| IBIS file nevis_100lqfp_derated.ibs generated by Daphne version: 2018.03.27
[IBIS Ver]   5.0
[Comment Char]   |_char
[File Name]   nevis_100lqfp_derated.ibs
[File Rev]   1
[Date]   Tue Nov  6 17:26:38 2018
[Source]   NXP Viper 2018.03.27
[Notes]
[Disclaimer] IMPORTANT NOTICE
  This information is provided on an AS IS basis and without warranty.
  IN NO EVENT SHALL NXP BE LIABLE FOR INCIDENTAL OR CONSEQUENTIAL
  DAMAGES ARISING FROM USE OF THIS INFORMATION. THIS DISCLAIMER OF
  WARRANTY EXTENDS TO THE USER OF THE INFORMATION, AND TO THEIR CUSTOMERS
  OR USERS OF PRODUCTS  AND IS IN LIEU OF ALL WARRANTIES WHETHER EXPRESS,
  IMPLIED, OR STATUTORY, INCLUDING IMPLIED WARRANTIES OF MERCHANTABILITY
  OR FITNESS FOR PARTICULAR PURPOSE.
  NXP does not represent or warrant that the information furnished
  hereunder is free of infringement of any third party patents,
  copyrights, trade secrets, or other intellectual property rights.
  NXP does not represent or warrant that the information is free of
  defect, or that it meets any particular standard, requirements or need
  of the user of the infomation or their customers.
  NXP reserves the right to change the information in this file
  without notice.
   http://www.nxp.com
[Copyright]   (C) Copyright NXP 2004 - 2018, All Rights Reserved.
|   NEVIS:100LQFP
[Component]   NEVIS:100LQFP
[Manufacturer]   NXP
[Package]
| variable   typ   min   max
R_pkg   0.12938   0.084596   0.14923
L_pkg   4.494e-09   3.339e-09   5.624e-09
C_pkg   9.253e-13   7.884e-13   1.210e-12
[Pin] signal_name   model_name   R_pin   L_pin   C_pin
1   TCK   p_io_5vtol_4m   0.13839   5.358e-09 9.081e-13
2   RESETB   p_vpp_5vtol_4m   0.084596  4.716e-09 1.210e-12
3   GPIOC0   p_io_5vtol_4m   0.12944   4.882e-09 9.510e-13
4   GPIOC1   p_io_5vtol_4m   0.12633   4.637e-09 9.568e-13
5   GPIOC2   p_io_5vtol_4m   0.12482   4.358e-09 9.723e-13
6   GPIOF8   p_io_5vtol_4m   0.12996   3.587e-09 8.978e-13
7   VDD33   POWER   NA   NA   NA
8   VSS   GND   NA   NA   NA
9   GPIOD6   p_io_5vtol_4m   0.12568   3.453e-09 8.861e-13
10   GPIOD5   p_io_5vtol_4m   0.12166   3.927e-09 8.389e-13
11   GPIOC3   p_io_5vtol_4m   0.11505   3.887e-09 8.150e-13
12   GPIOC4   p_io_5vtol_4m   0.11662   3.982e-09 9.402e-13
13   GPIOA10   p_io_5vtol_4m   0.11619   3.798e-09 7.884e-13
14   GPIOA9   p_io_5vtol_4m   0.12215   3.545e-09 8.020e-13
15   VSS   GND   NA   NA   NA
16   VDD   POWER   NA   NA   NA
17   GPIOA7   p_io_5vtol_4m   0.12328   3.627e-09 8.876e-13
18   GPIOA8   p_io_5vtol_4m   0.12024   4.091e-09 8.720e-13
19   GPIOA6   p_io_5vtol_4m   0.12076   4.379e-09 8.539e-13
20   GPIOA5   p_io_5vtol_4m   0.12153   4.556e-09 9.300e-13
21   GPIOA4   p_io_5vtol_4m   0.12459   4.784e-09 9.582e-13
22   GPIOA0   p_io_5vtol_4m   0.1277   4.982e-09 1.043e-12
23   GPIOA1   p_io_5vtol_4m   0.13134   5.169e-09 9.858e-13
24   GPIOA2   p_io_5vtol_4m   0.13511   5.278e-09 1.058e-12
25   GPIOA3   p_io_5vtol_4m   0.1403   5.579e-09 9.224e-13
26   GPIOB7   p_io_5vtol_4m   0.14428   5.567e-09 8.922e-13
27   GPIOC5   p_io_5vtol_4m   0.086695  4.756e-09 1.146e-12
28   GPIOB6   p_io_5vtol_4m   0.13488   4.874e-09 9.254e-13
29   GPIOB5   p_io_5vtol_4m   0.13539   4.494e-09 9.544e-13
30   GPIOB4   p_io_5vtol_4m   0.14179   3.764e-09 1.043e-12
31   VDDA   POWER   NA   NA   NA
32   VSSA   GND   NA   NA   NA
33   GPIOB0   p_io_5vtol_4m   0.13966   3.558e-09 8.476e-13
34   GPIOB1   p_io_5vtol_4m   0.14138   3.454e-09 8.946e-13
35   VDD   POWER   NA   NA   NA
36   GPIOB2   p_io_5vtol_4m   0.13932   3.570e-09 8.125e-13
37   GPIOA11   p_io_5vtol_4m   0.14249   3.673e-09 9.251e-13
38   VSS_USB   GND   NA   NA   NA
39   USB_DP   NC   0.14676   3.468e-09 8.492e-13
40   USB_DM   NC   0.14622   3.418e-09 9.220e-13
41   VDD_USB   POWER   NA   NA   NA
42   GPIOB3   p_io_5vtol_4m   0.14251   3.392e-09 8.778e-13
43   VDD33   POWER   NA   NA   NA
44   VSS   GND   NA   NA   NA
45   GPIOF11   p_io_5vtol_4m   0.14188   3.731e-09 9.937e-13
46   GPIOF15   p_io_5vtol_4m   0.13496   4.493e-09 9.338e-13
47   GPIOD7   p_io_5vtol_4m   0.13493   4.834e-09 1.059e-12
48   GPIOG11   p_io_5vtol_4m   0.13554   5.103e-09 9.630e-13
49   GPIOC6   p_io_5vtol_4m   0.13844   5.328e-09 1.077e-12
50   GPIOC7   p_io_5vtol_4m   0.14231   5.624e-09 9.638e-13
51   GPIOG10   p_io_5vtol_4m   0.1376   5.575e-09 9.335e-13
52   GPIOC8   p_io_5vtol_4m   0.12912   5.293e-09 1.144e-12
53   GPIOC9   p_io_5vtol_4m   0.12493   5.103e-09 9.020e-13
54   GPIOC10   p_io_5vtol_4m   0.12177   4.924e-09 9.088e-13
55   GPIOF0   p_io_5vtol_4m   0.11876   4.771e-09 9.386e-13
56   GPIOF10   p_io_5vtol_4m   0.1159   4.642e-09 9.030e-13
57   GPIOF9   p_io_5vtol_4m   0.11553   4.566e-09 9.000e-13
58   GPIOC11   p_io_5vtol_4m   0.11627   4.472e-09 8.361e-13
59   GPIOC12   p_io_5vtol_4m   0.11483   4.368e-09 8.595e-13
60   GPIOF2   p_io_5vtol_4m   0.1176   4.372e-09 8.162e-13
61   GPIOF3   p_io_5vtol_4m   0.11313   4.189e-09 8.385e-13
62   GPIOF4   p_io_5vtol_4m   0.11588   4.167e-09 8.970e-13
63   GPIOF5   p_io_5vtol_4m   0.11563   4.018e-09 8.227e-13
64   GPIOG8   p_io_5vtol_4m   0.11982   3.863e-09 8.749e-13
65   GPIOG9   p_io_5vtol_4m   0.12628   3.339e-09 8.566e-13
66   VSS   GND   NA   NA   NA
67   VDD33   POWER   NA   NA   NA
68   GPIOE0   p_io_5vtol_4m   0.12511   3.377e-09 8.919e-13
69   GPIOE1   p_io_5vtol_4m   0.12114   3.994e-09 9.443e-13
70   GPIOG2   p_io_5vtol_4m   0.11972   4.420e-09 8.645e-13
71   GPIOG3   p_io_5vtol_4m   0.12202   4.650e-09 9.264e-13
72   GPIOE8   p_io_5vtol_4m   0.12507   4.855e-09 9.863e-13
73   GPIOE9   p_io_5vtol_4m   0.12842   5.115e-09 9.686e-13
74   GPIOE2   p_io_5vtol_4m   0.13118   5.146e-09 1.158e-12
75   GPIOE3   p_io_5vtol_4m   0.13753   5.584e-09 9.666e-13
76   GPIOC13   p_io_5vtol_4m   0.13853   5.575e-09 8.947e-13
77   GPIOF1   p_io_5vtol_4m   0.13496   5.359e-09 1.077e-12
78   GPIOG0   p_io_5vtol_4m   0.13315   5.306e-09 9.438e-13
79   GPIOG1   p_io_5vtol_4m   0.13136   5.158e-09 9.924e-13
80   GPIOG4   p_io_5vtol_4m   0.12979   5.044e-09 9.827e-13
81   GPIOG5   p_io_5vtol_4m   0.12816   4.901e-09 9.434e-13
82   GPIOE4   p_io_5vtol_4m   0.12859   4.863e-09 9.887e-13
83   GPIOE5   p_io_5vtol_4m   0.12817   4.776e-09 8.692e-13
84   GPIOE6   p_io_5vtol_4m   0.12806   4.701e-09 8.519e-13
85   GPIOE7   p_io_5vtol_4m   0.13011   4.532e-09 8.129e-13
86   GPIOG6   p_io_5vtol_4m   0.12685   4.408e-09 8.755e-13
87   GPIOC14   p_io_5vtol_4m   0.13081   4.541e-09 8.955e-13
88   GPIOC15   p_io_5vtol_4m   0.13031   4.390e-09 7.979e-13
89   GPIOF12   p_io_5vtol_4m   0.13395   4.507e-09 8.889e-13
90   GPIOF13   p_io_5vtol_4m   0.13488   4.459e-09 8.414e-13
91   GPIOF14   p_io_5vtol_4m   0.14287   4.481e-09 8.031e-13
92   GPIOG7   p_io_5vtol_4m   0.14833   4.048e-09 8.642e-13
93   VDD   POWER   NA   NA   NA
94   GPIOF6   p_io_5vtol_4m   0.14823   3.872e-09 8.742e-13
95   GPIOF7   p_io_5vtol_4m   0.14688   3.915e-09 9.017e-13
96   VDD33   POWER   NA   NA   NA
97   VSS   GND   NA   NA   NA
98   TDO   p_io_5vtol_4m   0.14923   4.080e-09 9.835e-13
99   TMS   p_io_5vtol_4m   0.14208   4.773e-09 1.036e-12
100   TDI   p_io_5vtol_4m   0.14429   5.291e-09 9.163e-13
101   NC   NC   NA   NA   NA
[Pin Mapping]   pulldown_ref   pullup_ref
1   NC   NC
2   NC   NC
3   NC   NC
4   NC   NC
5   NC   NC
6   NC   NC
7   NC   VDD33
8   VSS   NC
9   NC   NC
10   NC   NC
11   NC   NC
12   NC   NC
13   NC   NC
14   NC   NC
15   VSS   NC
16   NC   VDD
17   NC   NC
18   NC   NC
19   NC   NC
20   NC   NC
21   NC   NC
22   NC   NC
23   NC   NC
24   NC   NC
25   NC   NC
26   NC   NC
27   NC   NC
28   NC   NC
29   NC   NC
30   NC   NC
31   NC   VDDA
32   VSSA   NC
33   NC   NC
34   NC   NC
35   NC   VDD
36   NC   NC
37   NC   NC
38   VSS_USB   NC
39   NC   NC
40   NC   NC
41   NC   VDD_USB
42   NC   NC
43   NC   VDD33
44   VSS   NC
45   NC   NC
46   NC   NC
47   NC   NC
48   NC   NC
49   NC   NC
50   NC   NC
51   NC   NC
52   NC   NC
53   NC   NC
54   NC   NC
55   NC   NC
56   NC   NC
57   NC   NC
58   NC   NC
59   NC   NC
60   NC   NC
61   NC   NC
62   NC   NC
63   NC   NC
64   NC   NC
65   NC   NC
66   VSS   NC
67   NC   VDD33
68   NC   NC
69   NC   NC
70   NC   NC
71   NC   NC
72   NC   NC
73   NC   NC
74   NC   NC
75   NC   NC
76   NC   NC
77   NC   NC
78   NC   NC
79   NC   NC
80   NC   NC
81   NC   NC
82   NC   NC
83   NC   NC
84   NC   NC
85   NC   NC
86   NC   NC
87   NC   NC
88   NC   NC
89   NC   NC
90   NC   NC
91   NC   NC
92   NC   NC
93   NC   VDD
94   NC   NC
95   NC   NC
96   NC   VDD33
97   VSS   NC
98   NC   NC
99   NC   NC
100   NC   NC
101   NC   NC
|*   Model Selector   *
[Model Selector] p_io_5vtol_4m
p_io_5vtol_4m_dse1_sre0   io, full drive mode without slew rate
p_io_5vtol_4m_dse1_sre1   io, full drive mode with slew rate
p_io_5vtol_4m_dse0_sre0   io, low drive mode without slew rate
p_io_5vtol_4m_dse0_sre1   io, low drive mode with slew rate
| End [Component] NEVIS:100LQFP
| Models and submodels in the file (5): p_io_5vtol_4m_dse0_sre0 (I/O), p_io_5vtol_4m_dse0_sre1 (I/O), p_io_5vtol_4m_dse1_sre0 (I/O), p_io_5vtol_4m_dse1_sre1 (I/O), p_vpp_5vtol_4m (I/O_open_drain)
